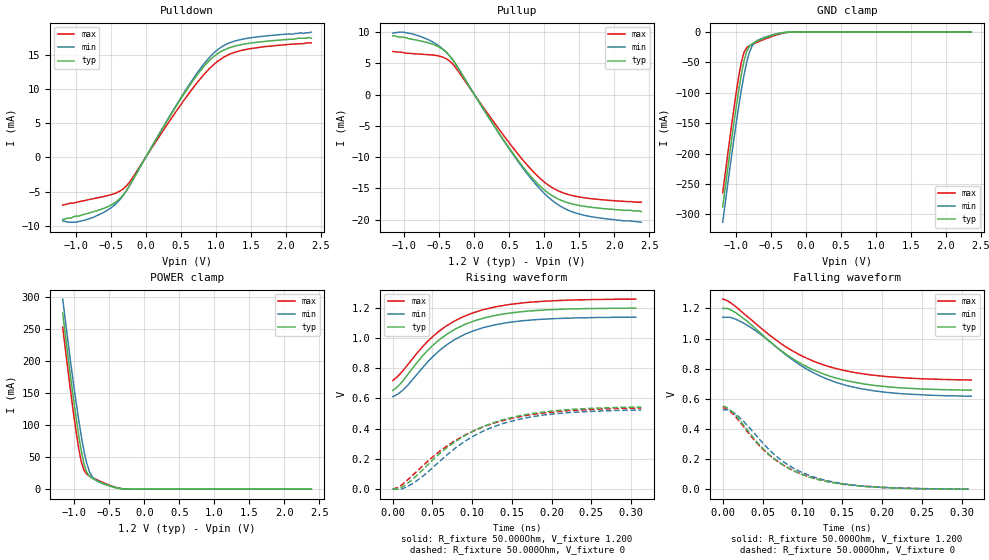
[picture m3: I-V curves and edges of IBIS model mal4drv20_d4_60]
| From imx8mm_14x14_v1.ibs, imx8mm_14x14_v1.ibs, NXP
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[Model] mal4drv20_d4_60
Model_type   I/O
Polarity   Non-Inverting
Enable   Active-High
C_comp   1.691pF   1.683pF   1.699pF
C_comp_pullup   737.671fF   724.063fF   743.649fF
C_comp_pulldown 903.204fF   890.383fF   921.747fF
Vinh = 924.000mV
Vinl = 809.000mV
Vmeas = 867.000mV
Vref = 867.000mV
Rref = 50Ohms
Cref = 0pF
[Model Spec]
Vinh   924.000mV   881.000mV   968.000mV
Vinl   809.000mV   766.000mV   853.000mV
Vmeas   867.000mV   823.000mV   910.000mV
Vref   867.000mV   823.000mV   910.000mV
D_overshoot_ampl_h 0.24 NA   NA
D_overshoot_ampl_l 0.24 NA   NA
D_overshoot_area_l 300.000m NA   NA
D_overshoot_area_h 300.000m NA   NA
|[Receiver Thresholds]
|Vth = 867.000mV
|Vth_min = 823.000mV
|Vth_max = 910.000mV
|Vinh_ac = 68.000mV
|Vinh_dc = 68.000mV
|Vinl_ac = -68.000mV
|Vinl_dc = -68.000mV
|Tslew_ac = 5.000ns
|Threshold_sensitivity = 0.5
|Reference_supply Pullup_ref
[Temperature Range]   25.000   125.000   -40.000
[Voltage Range]   1.200V   1.140V   1.260V
[GND Clamp Reference]   0.00V   0.00V   0.00V
|[C Comp Corner]
|| variable   typ   min   max
|C_comp 1.699pF   1.683pF   1.691pF
|C_comp_pullup 743.649fF   724.063fF   737.671fF
|C_comp_pulldown 903.204fF   921.747fF   890.383fF
[Pulldown Reference]   0.00V   0.00V   0.00V
[POWER Clamp Reference]   1.200V   1.140V   1.260V
[Pullup Reference]   1.200V   1.140V   1.260V
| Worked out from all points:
|   slope of the pulldown table from 0 to 0.18 V, typ, clamps not added: 56.8 ohm
|   slope of the pullup table from 0 to 0.18 V, typ, clamps not added: 56.2 ohm
|   GND clamp passes 1 mA (typ) near -0.33 V on its own axis
|   POWER clamp passes 1 mA (typ) near -0.36 V on its own axis
|   rising waveform, R_fixture 50.000Ohm, V_fixture 1.200: 20-80 % time 70.9ps typ, 70.9ps min, 73.5ps max; typ from 0.653 V to 1.2 V
|   rising waveform, R_fixture 50.000Ohm, V_fixture 0: 20-80 % time 90.2ps typ, 88ps min, 94.9ps max; typ from -0.002 V to 0.543 V
|   falling waveform, R_fixture 50.000Ohm, V_fixture 1.200: 20-80 % time 90.1ps typ, 90.1ps min, 93.7ps max; typ from 1.2 V to 0.658 V
|   falling waveform, R_fixture 50.000Ohm, V_fixture 0: 20-80 % time 69.7ps typ, 70.8ps min, 71.7ps max; typ from 0.549 V to 0.001 V
[GND Clamp]
-1.184V   -287.4mA   -312.7mA   -264.2mA
-1.031V   -155.3mA   -181.5mA   -131.2mA
-954.6mV  -95.39mA   -121.7mA   -72.46mA
-916.4mV  -69mA      -94.39mA   -48.75mA
-878.2mV  -46.95mA   -69.72mA   -32.79mA
-840mV    -31.44mA   -48.8mA    -25.56mA
-801.8mV  -23.08mA   -32.94mA   -22.5mA
-763.6mV  -19.1mA    -22.7mA    -20.38mA
-725.5mV  -16.66mA   -16.96mA   -18.44mA
-496.4mV  -6.091mA   -5.301mA   -7.811mA
-229.1mV  -85.34uA   -131.6uA   -211.4uA
2.367V    74.27nA    1.057uA    27.11nA
[Power Clamp]
-1.167V   274.5mA    296.4mA    252.6mA
-1.015V   142.4mA    166mA      119.9mA
-938.2mV  83.72mA    107.6mA    63.18mA
-900mV    58.71mA    81.52mA    42.14mA
-861.8mV  39mA       58.71mA    29.24mA
-823.6mV  26.53mA    40.39mA    23.35mA
-785.5mV  20.35mA    27.47mA    20.48mA
-747.3mV  17.16mA    19.6mA     18.3mA
-709.1mV  14.88mA    15.15mA    16.26mA
-480mV    4.411mA    4.49mA     5.397mA
-250.9mV  59.97uA    214.6uA    73.54uA
2.384V    -51.61nA   -1.045uA   -11.93nA
[Pulldown]
-1.184V   -9.1mA     -9.3mA     -7mA
-992.7mV  -8.6mA     -9.5mA     -6.6mA
-801.8mV  -8.14mA    -8.98mA    -6.17mA
-572.7mV  -7.366mA   -7.91mA    -5.66mA
-381.8mV  -6.174mA   -6.363mA   -5.015mA
-229.1mV  -4.099mA   -4.144mA   -3.616mA
649.1mV   10.86mA    11.09mA    9.816mA
840mV     13.44mA    13.82mA    12.25mA
1.031V    15.25mA    15.83mA    14.13mA
1.184V    16.05mA    16.76mA    15.08mA
1.451V    16.71mA    17.48mA    15.89mA
2.367V    17.5mA     18.4mA     16.8mA
[Pullup]
-1.167V   9.4mA      9.814mA    6.9mA
-1.015V   9.2mA      10mA       6.714mA
-709.1mV  8.42mA     9.027mA    6.421mA
-480mV    7.449mA    7.558mA    6.092mA
-327.3mV  5.853mA    5.823mA    5.103mA
207.3mV   -3.676mA   -3.728mA   -3.296mA
550.9mV   -9.392mA   -9.55mA    -8.49mA
818.2mV   -13.23mA   -13.56mA   -12.06mA
1.047V    -15.67mA   -16.31mA   -14.39mA
1.276V    -17.07mA   -18.14mA   -15.74mA
1.505V    -17.74mA   -19.12mA   -16.38mA
2.384V    -18.7mA    -20.4mA    -17.2mA
[Ramp]
R_load=50.000Ohm
dV/dt_r   328.050mV/82.500ps  316.047mV/81.500ps  323.910mV/86.500ps
dV/dt_f   328.050mV/82.000ps  316.048mV/82.500ps  323.910mV/84.500ps
[Rising waveform]
R_fixture=50.000Ohm
V_fixture=1.200
V_fixture_min=1.140
V_fixture_max=1.260
0s        652.8mV    611.8mV    718.9mV
8ps       687.6mV    634.7mV    755.6mV
17ps      744.8mV    676.4mV    810.5mV
37ps      878.1mV    800.3mV    939.4mV
54ps      968.6mV    894.6mV    1.026V
75ps      1.048V     980.2mV    1.105V
104ps     1.117V     1.052V     1.172V
129ps     1.15V      1.089V     1.207V
176ps     1.181V     1.121V     1.239V
306ps     1.199V     1.139V     1.259V
[Rising waveform]
R_fixture=50.000Ohm
V_fixture=0
0s        -2.331mV   -1.886mV   -1.237mV
9ps       2.807mV    -1.886mV   16.01mV
27ps      72.58mV    41.5mV     99.53mV
55ps      214.9mV    162.5mV    232mV
79ps      314.3mV    270.8mV    320.9mV
110ps     404.1mV    373.1mV    402.8mV
136ps     454.4mV    428.5mV    449mV
167ps     491.6mV    470mV      486mV
196ps     513.7mV    493.3mV    506.4mV
313ps     542.7mV    522.8mV    536mV
[Falling waveform]
R_fixture=50.000Ohm
V_fixture=1.200
V_fixture_min=1.140
V_fixture_max=1.260
0s        1.2V       1.141V     1.262V
10ps      1.191V     1.14V      1.237V
30ps      1.117V     1.091V     1.15V
80ps      894.2mV    888.9mV    942.7mV
104ps     817.7mV    801.5mV    872.6mV
127ps     764.2mV    739.6mV    824.5mV
156ps     719.7mV    687.8mV    784.4mV
190ps     689.5mV    653.1mV    756.3mV
239ps     668.3mV    629.2mV    735.8mV
312ps     657.6mV    617.5mV    724.9mV
[Falling waveform]
R_fixture=50.000Ohm
V_fixture=0
0s        549.1mV    528.1mV    542mV
7ps       536.4mV    526.1mV    525.5mV
19ps      474.4mV    487mV      464.3mV
41ps      325.8mV    362.9mV    317.8mV
63ps      210.3mV    239.5mV    207.8mV
81ps      145.3mV    165.2mV    145.3mV
108ps     82.18mV    93.98mV    84.59mV
139ps     42.66mV    48.24mV    44.94mV
181ps     17.52mV    19.81mV    19.22mV
309ps     1.158mV    1.316mV    1.383mV
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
